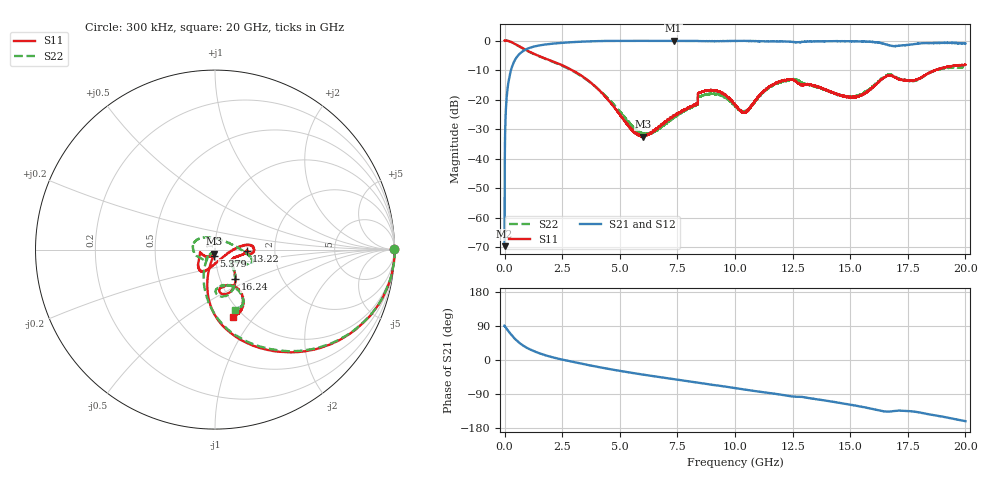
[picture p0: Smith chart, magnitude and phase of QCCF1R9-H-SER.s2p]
!QCCF1R9
!Johanson Technology Inc.
!www.johansontechnology.com
!Test Board Conditions:
!Substrate Type  RO4350B
!Substrate Thickness  10 mil
!Substrate Dk  3.66
!TL Type: GCPW
!TL Trace Width  21 mil
!TL Gap  20 mil
!Electrode orientation  Horizontal
!DUT TOPOLOGY	SERIES
!Mounting Pad LxW  16x21 mil
# MHz S  dB  R 50
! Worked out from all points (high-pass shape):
!   20001 points, 300 kHz to 20 GHz, reference 50 ohm
!   highest |S21| = -0.10 dB at 7.332 GHz (marker M1); lowest = -69.7 dB at 300 kHz (marker M2)
!   |S21| within 3 dB of the highest: 907.7 MHz to end of sweep
!   lowest |S11| = -32.5 dB at 6.01 GHz (marker M3), VSWR 1.05, Z = 49.7 - j2.32 ohm
!   |S11| at or under -10 dB: 2.925 GHz to 18.71 GHz (15.78 GHz wide, 146 % of centre); 18.70864 GHz to 18.70938 GHz (735 kHz wide, 0.00393 % of centre)
!   |S22| runs from -31.9 to 0.0 dB; largest |S21 - S12| = 0.03
!   S11 on the Smith chart (normalised r, x): 300 kHz: open; 5.379 GHz: 0.98, -0.07; 13.22 GHz: 1.43, -0.03; 16.24 GHz: 1.18, -0.40; 20 GHz: 0.90, -0.79
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0.3  -0.03 0.1  -69.72 90.4  -67.94 90.8  -0.04 0.0
101.298  -0.06 -8.2  -18.25 81.5  -18.27 81.6  -0.05 -8.3
126.298  -0.09 -10.2  -16.38 79.5  -16.40 79.6  -0.09 -10.3
248.296  -0.39 -19.6  -10.86 69.8  -10.87 70.0  -0.39 -19.7
450.293  -1.14 -33.2  -6.59 55.8  -6.58 56.0  -1.18 -33.4
1480.278  -5.21 -71.2  -1.71 18.4  -1.70 18.2  -5.27 -70.6
3334.25  -11.90 -98.9  -0.40 -9.8  -0.40 -9.7  -12.11 -102.2
5379.219  -28.91 -103.2  -0.12 -32.5  -0.12 -32.5  -27.48 -134.7
6010.21  -32.55 -97.1  -0.12 -38.6  -0.12 -38.5  -31.69 -136.4
6667.2  -29.57 -110.0  -0.12 -44.6  -0.12 -44.5  -30.09 -136.4
7332.19  -25.54 -130.1  -0.10 -50.6  -0.12 -50.5  -26.13 -136.3
8763.169  -17.12 -128.4  -0.20 -63.2  -0.20 -63.2  -18.38 -179.8
10000.15  -21.66 -92.4  -0.14 -74.1  -0.16 -73.9  -22.25 120.9
10481.14  -24.20 -37.8  -0.16 -78.6  -0.14 -78.2  -23.99 61.0
12078.12  -13.70 5.1  -0.31 -92.4  -0.34 -92.6  -13.96 -11.5
13224.1  -15.05 -3.1  -0.31 -100.6  -0.34 -100.4  -15.09 -22.4
13334.1  -15.18 -4.6  -0.32 -101.6  -0.34 -101.7  -15.24 -22.6
15125.07  -19.21 -33.2  -0.22 -119.3  -0.27 -119.4  -19.08 -37.0
16243.06  -14.03 -55.0  -0.72 -132.9  -0.72 -133.1  -13.76 -56.6
16667.05  -11.93 -73.6  -1.59 -136.2  -1.58 -136.9  -11.53 -76.6
17773.03  -13.54 -70.5  -1.23 -136.2  -1.24 -136.6  -13.64 -74.0
20000  -8.23 -74.9  -1.02 -161.3  -0.85 -160.0  -9.01 -71.6
